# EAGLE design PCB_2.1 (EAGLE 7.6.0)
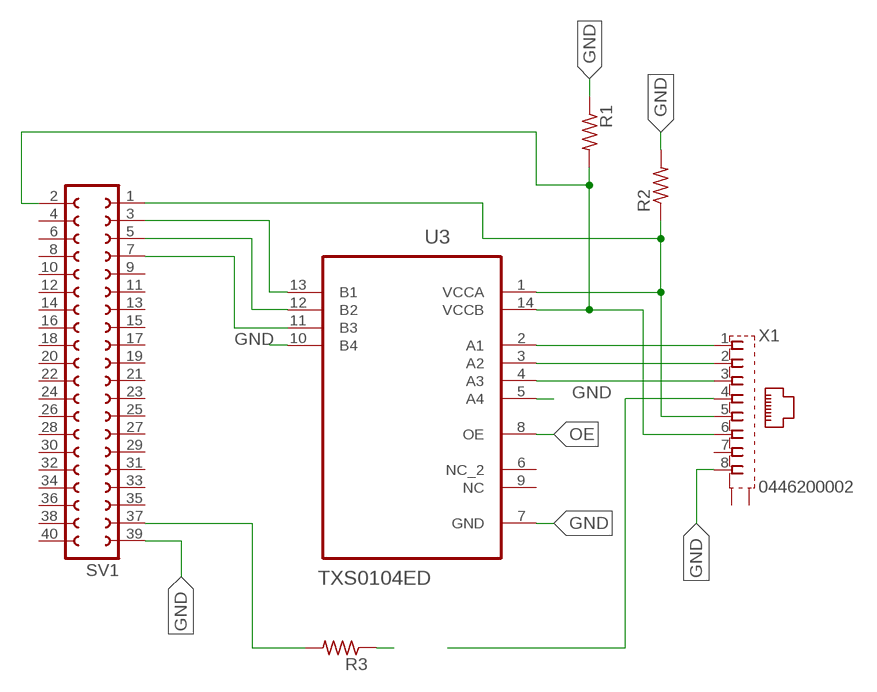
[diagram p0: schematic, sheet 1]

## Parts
R1  R-US_R0805  [R0805]
R2  R-US_R0805  [R0805]
R3  R-US_R0805  [R0805]
SV1  FE20-2  [FE20-2]
U3  TXS0104ED  [SOIC127P600X175-14N]
X1  0446200002  [0446200002]

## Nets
A1: U3.2(A1) X1.1
A2: U3.3(A2) X1.2
A3: U3.4(A3) X1.3
GND: R1.1 R2.2 SV1.39 U3.5(A4) U3.7(GND) U3.10(B4) X1.8
INT: SV1.7 U3.11(B3)
LED: X1.4
N$1: R3.2 SV1.37
N$2: R3.1
OE: U3.8(OE)
SCL: SV1.5 U3.12(B2)
SDA: SV1.3 U3.13(B1)
VCCA: R2.1 SV1.1 U3.1(VCCA) X1.5
VCCB: R1.2 SV1.2 U3.14(VCCB) X1.6
Unconnected: SV1.4 SV1.6 SV1.8 SV1.9 SV1.10 SV1.11 SV1.12 SV1.13 SV1.14 SV1.15 SV1.16 SV1.17 SV1.18 SV1.19 SV1.20 SV1.21 SV1.22 SV1.23 SV1.24 SV1.25 SV1.26 SV1.27 SV1.28 SV1.29 SV1.30 SV1.31 SV1.32 SV1.33 SV1.34 SV1.35 SV1.36 SV1.38 SV1.40 U3.6(NC_2) U3.9(NC) X1.7 X1.S@1(S1) X1.S@2(S2)

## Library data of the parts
R1-R3 = resistor:R-US_: RESISTOR, American symbol
SV1 = con-lsta:FE20-2: FEMALE HEADER; OC_FARNELL: unknown; OC_NEWARK: unknown
U3 = TXS0104ED:TXS0104ED: 4-BIT BIDIRECTIONAL VOLTAGE-LEVEL TRANSLATOR FOR OPEN-DRAIN AND PUSH-PULL APPLICATIONS; AVAILABILITY: Unavailable; DESCRIPTION: 4-Bit Bidirectional Voltage-Level Shifter for Open-Drain and Push-Pull Applications 14-SOIC -40 to 85; MF: Texas Instruments; MP: TXS0104ED; PACKAGE: SOIC-14 Texas Instruments; PRICE: None
X1 = 0446200002:0446200002: RJ-45 INVERTED MODULAR JACK ASSEMBLY WITH RJ-11 KEEPOUT FEATURE Source: Data sheet MOLEX 0446200002 BUCHSE, RJ45, GESCHIRMT Source: Farnell; AVAILABILITY: Unavailable; DESCRIPTION: Conn RJ-45 RCP 8 POS 2.04mm Solder RA Thru-Hole 8 Terminal 1 Port Tray Cat 3; MF: Molex, LLC; MP: 0446200002; PACKAGE: None; PRICE: None

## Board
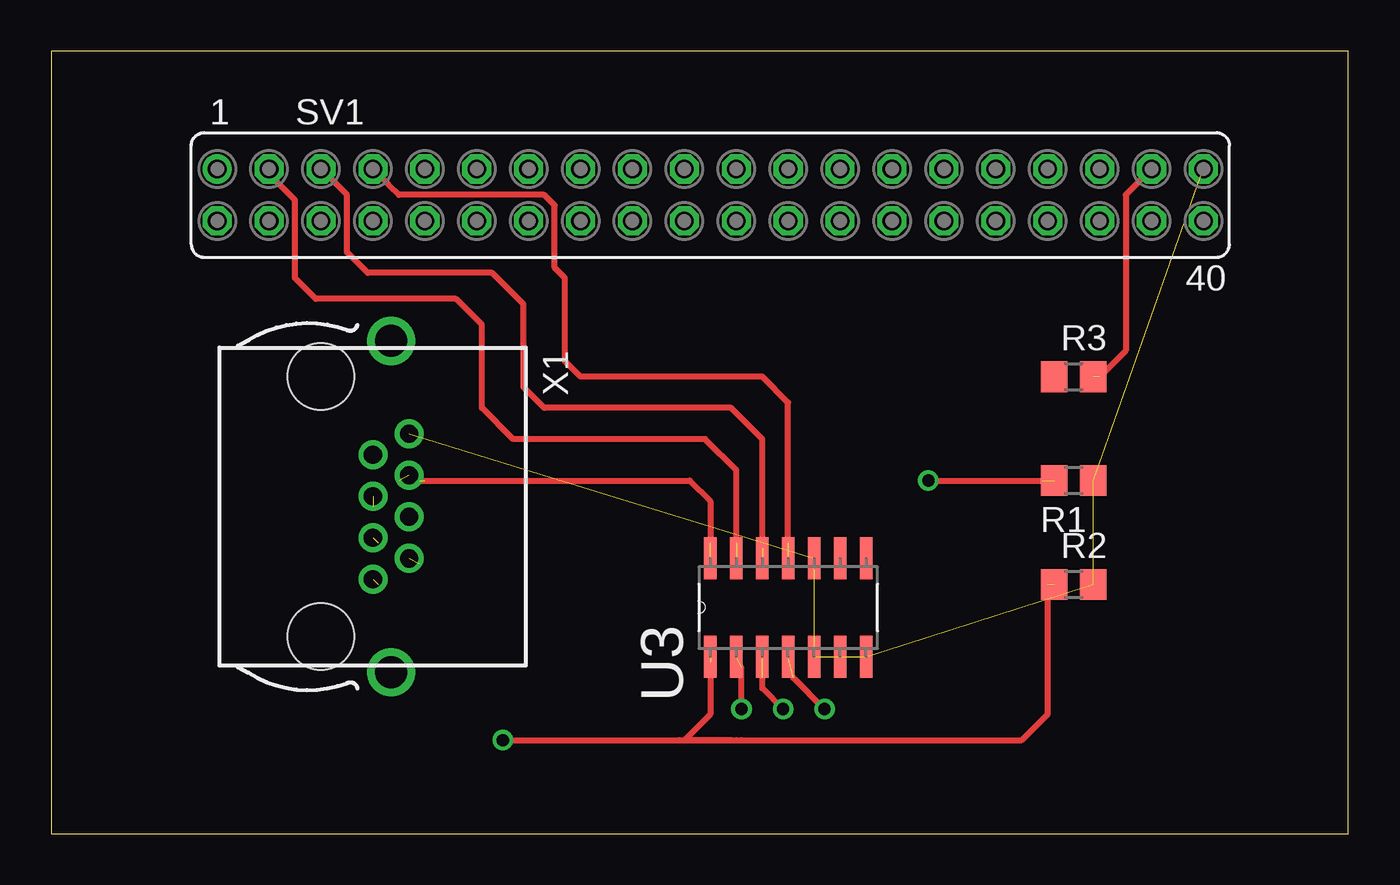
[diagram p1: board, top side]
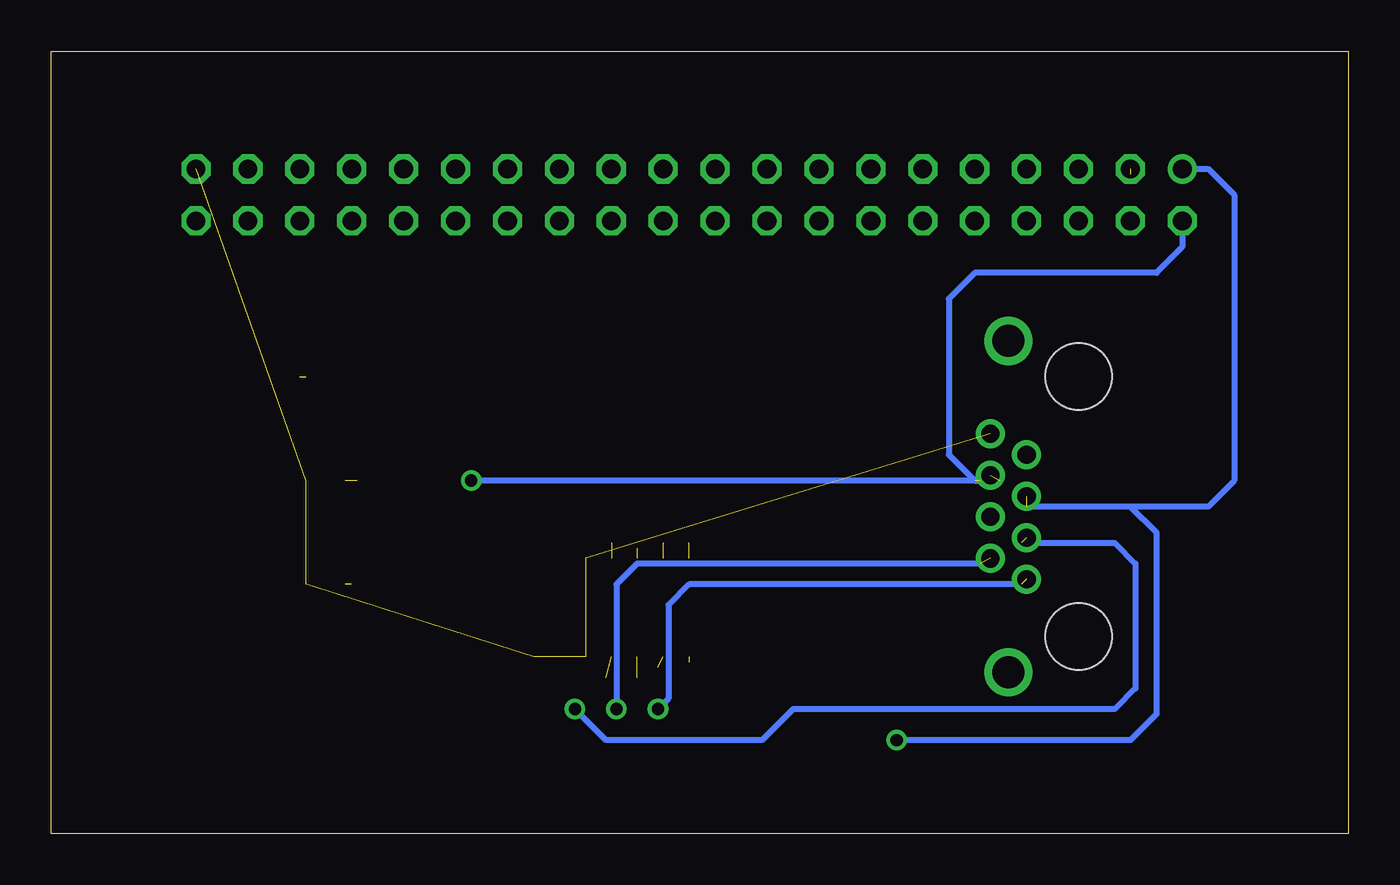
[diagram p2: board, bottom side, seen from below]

Size 63.48 x 38.28 mm. Coordinates in mm from the lower left corner, seen from the top.
Outline: 0,0 63.48,0 63.48,38.28 0,38.28 0,0
Copper layers (1*16): Top 0.035mm / dielectric 1.5mm / Bottom 0.035mm
Design rules "default *": minimum track width 10mil, minimum drill 24mil, track to track 8mil, track to pad 8mil, pad to pad 8mil, via to via 8mil, smd to smd 8mil, copper to edge 20mil, drill to drill 8mil, minimum pad ring 10mil, minimum via ring 8mil, stop-mask expansion 4mil, vias tented up to drill 0mil, thermal gap 10mil

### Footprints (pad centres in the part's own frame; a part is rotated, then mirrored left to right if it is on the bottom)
R0805 = smd 1.3 x 1.5: 1 -0.95,0; 2 0.95,0
FE20-2 = drill 0.914: 1 -24.13,1.27 | drill 0.914 octagon: 2 -24.13,-1.27; 3 -21.59,1.27; 4 -21.59,-1.27; 5 -19.05,1.27; 6 -19.05,-1.27; 7 -16.51,1.27; 8 -16.51,-1.27; 9 -13.97,1.27; 10 -13.97,-1.27; 11 -11.43,1.27; 12 -11.43,-1.27; 13 -8.89,1.27; 14 -8.89,-1.27; 15 -6.35,1.27; 16 -6.35,-1.27; 17 -3.81,1.27; 18 -3.81,-1.27; 19 -1.27,1.27; 20 -1.27,-1.27; 21 1.27,1.27; 22 1.27,-1.27; 23 3.81,1.27; 24 3.81,-1.27; 25 6.35,1.27; 26 6.35,-1.27; 27 8.89,1.27; 28 8.89,-1.27; 29 11.43,1.27; 30 11.43,-1.27; 31 13.97,1.27; 32 13.97,-1.27; 33 16.51,1.27; 34 16.51,-1.27; 35 19.05,1.27; 36 19.05,-1.27; 37 21.59,1.27; 38 21.59,-1.27; 39 24.13,1.27; 40 24.13,-1.27
SOIC127P600X175-14N = smd 2.057 x 0.61: 1 -4.801,7.62; 2 -4.801,6.35; 3 -4.801,5.08; 4 -4.801,3.81; 5 -4.801,2.54; 6 -4.801,1.27; 7 -4.801,0; 8 0,0; 9 0,1.27; 10 0,2.54; 11 0,3.81; 12 0,5.08; 13 0,6.35; 14 0,7.62
0446200002 = drill 0.889 pad 1.422: 1 3.556,2.54; 2 2.54,4.318; 3 1.524,2.54; 4 0.508,4.318; 5 -0.508,2.54; 6 -1.524,4.318; 7 -2.54,2.54; 8 -3.556,4.318 | drill 1.575 pad 2.286: S@1 -8.103,3.429; S@2 8.103,3.429 | hole 3.251: 6.35,0; -6.35,0

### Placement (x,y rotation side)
R1  50.04,17.27 180 top
R2  50.04,12.19 0 top
R3  50.04,22.35 0 top
SV1  32.26,31.24 0 top
U3  39.88,13.46 90 top
X1  13.21,16 270 top

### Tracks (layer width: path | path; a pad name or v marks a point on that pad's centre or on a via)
A1  (via drill 0.6)  (2 unrouted)
  Top 0.305: v33.78,6.1 33.78,8.13
  Bottom 0.305: 16,12.19 32.26,12.19 33.27,11.18 33.27,6.6 v33.78,6.1
A2  (via drill 0.6)  (2 unrouted)
  Top 0.305: v35.81,6.1 34.8,7.11 34.8,7.62
  Bottom 0.305: 18.03,13.21 34.8,13.21 35.81,12.19 v35.81,6.1
A3  (via drill 0.6)  (2 unrouted)
  Top 0.305: v37.85,6.1 36.32,7.62
  Bottom 0.305: 16,14.22 11.43,14.22 10.41,13.21 10.41,7.11 11.43,6.1 27.18,6.1 28.7,4.57 36.32,4.57 v37.85,6.1
GND  (6 unrouted)
INT  (1 unrouted)
  Top 0.305: 36.07,14.22 36.07,21.08 34.8,22.35 25.91,22.35 25.15,23.11 25.15,27.18 24.64,27.69 24.64,30.73 24.13,31.24 17.02,31.24 16.51,31.75 SV1.7
N$1  (1 unrouted)
  Top 0.305: SV1.37 52.58,31.24 52.58,23.62 51.31,22.35
SCL  (1 unrouted)
  Top 0.305: 34.8,13.97 34.8,19.3 33.27,20.83 24.13,20.83 23.11,21.84 23.11,25.91 21.59,27.43 15.49,27.43 14.48,28.45 14.48,31.24 SV1.5
SDA  (2 unrouted)
  Top 0.305: 33.53,14.22 33.53,17.78 32,19.3 22.61,19.3 21.08,20.83 21.08,24.89 19.81,26.16 12.95,26.16 11.94,27.18 11.94,30.99 10.67,32.26
VCCA  (via drill 0.6)  (3 unrouted)
  Top 0.305: v22.1,4.57 30.73,4.57 30.99,4.57 | 32.26,8.38 32.26,5.84 30.99,4.57 | 48.77,12.19 48.77,5.84 47.5,4.57 33.78,4.57 33.53,4.57 30.99,4.57 | 33.27,4.57 30.99,4.57
  Bottom 0.305: SV1.1 6.86,32.51 5.59,31.24 5.59,17.27 6.86,16 10.67,16 | 10.67,16 15.75,16 | 10.67,16 9.4,14.73 9.4,5.84 10.67,4.57 v22.1,4.57
VCCB  (via drill 0.6)  (4 unrouted)
  Top 0.305: v42.93,17.27 48.51,17.27 | 18.03,17.27 31.24,17.27 32.26,16.26 32.26,14.22
  Bottom 0.305: SV1.2 8.13,28.7 9.4,27.43 18.29,27.43 19.56,26.16 19.56,18.54 18.29,17.27 | 18.29,17.27 17.02,17.27 | 18.29,17.27 v42.93,17.27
